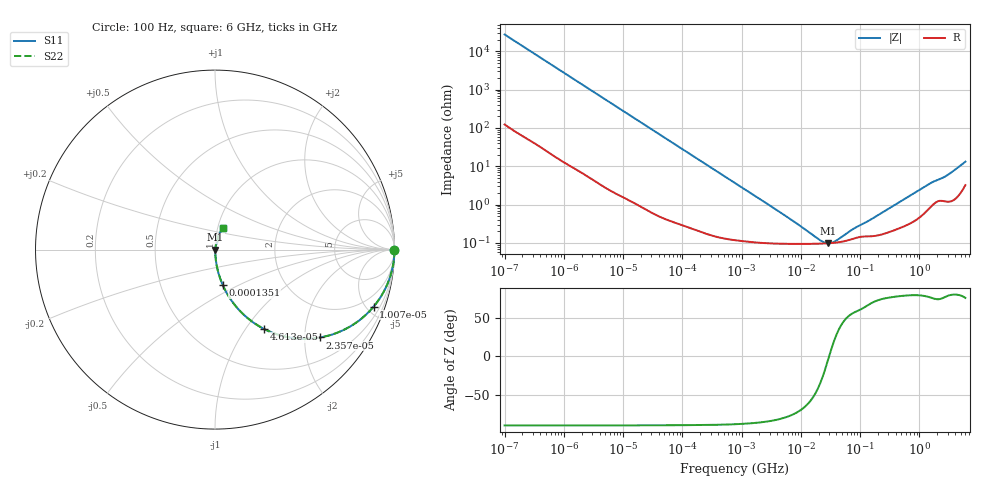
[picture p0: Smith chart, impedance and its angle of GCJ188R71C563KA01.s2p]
!Murata Part Number: GCJ188R71C563KA01
!These Parameters are Measured in Series Mode Connection
!Data Generated on Mar 13, 2026
!  o--ll--o
!Port1  Port2
!  o------o
!Operation Temp=25[degC], DC Bias Voltage=0[V]
!Freq. Start=100[Hz] Stop=6[GHz] 401[Steps]
# Hz S RI R 50
!Freq.(Hz) S11(Real) S11(Imag) S21(Real) S21(Imag) S12(Real) S12(Imag) S22(Real) S22(Imag)
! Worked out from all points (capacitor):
!   401 points, 100 Hz to 6 GHz, reference 50 ohm
!   read as one part in series: C = 57.6 nF near 109 Hz
!   lowest |Z| = 98.6 mohm at 29.12 MHz (marker M1)
!   series resonance near 30.04 MHz, so ESL is about 490 pH
!   S11 on the Smith chart (normalised r, x): 100 Hz: open; 10.07 kHz: 1.03, -5.55; 23.57 kHz: 1.02, -2.38; 46.13 kHz: 1.01, -1.22; 135.1 kHz: 1.00, -0.42; 6 GHz: 1.06, +0.26
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100  1 -0.00363  2.94e-05 0.00363  2.94e-05 0.00363  1 -0.00363
2008  0.9945 -0.0718  0.00553 0.0718  0.00553 0.0718  0.9945 -0.0718
4702  0.9716 -0.1637  0.0284 0.1637  0.0284 0.1637  0.9716 -0.1637
10066  0.8838 -0.3177  0.1162 0.3177  0.1162 0.3177  0.8838 -0.3177
15062  0.7741 -0.4152  0.2259 0.4152  0.2259 0.4152  0.7741 -0.4152
23569  0.5855 -0.4894  0.4145 0.4894  0.4145 0.4894  0.5855 -0.4894
40335  0.3277 -0.4658  0.6723 0.4658  0.6723 0.4658  0.3277 -0.4658
46134  0.2721 -0.4414  0.7279 0.4414  0.7279 0.4414  0.2721 -0.4414
75495  0.1243 -0.3254  0.8757 0.3254  0.8757 0.3254  0.1243 -0.3254
135116  0.044 -0.1993  0.956 0.1993  0.956 0.1993  0.044 -0.1993
289253  0.0111 -0.0968  0.9889 0.0968  0.9889 0.0968  0.0111 -0.0968
774597  0.00252 -0.0366  0.9975 0.0366  0.9975 0.0366  0.00252 -0.0366
5554849  0.000975 -0.00498  0.999 0.00498  0.999 0.00498  0.000975 -0.00498
1.555665e7  0.000952 -0.00135  0.999 0.00135  0.999 0.00135  0.000952 -0.00135
2.225763e7  0.000964 -0.000579  0.999 0.000579  0.999 0.000579  0.000964 -0.000579
2.911731e7  0.000983 -5.91e-05  0.999 5.91e-05  0.999 5.91e-05  0.000983 -5.91e-05
3.983537e7  0.00103 0.00054  0.999 -0.00054  0.999 -0.00054  0.00103 0.00054
7.797396e7  0.0013 0.00196  0.9987 -0.00196  0.9987 -0.00196  0.0013 0.00196
3.124326e8  0.00199 0.00788  0.998 -0.00788  0.998 -0.00788  0.00199 0.00788
1.431855e9  0.00863 0.0327  0.9914 -0.0327  0.9914 -0.0327  0.00863 0.0327
2.802721e9  0.0148 0.0528  0.9852 -0.0528  0.9852 -0.0528  0.0148 0.0528
6e9  0.0461 0.1185  0.9539 -0.1185  0.9539 -0.1185  0.0461 0.1185
